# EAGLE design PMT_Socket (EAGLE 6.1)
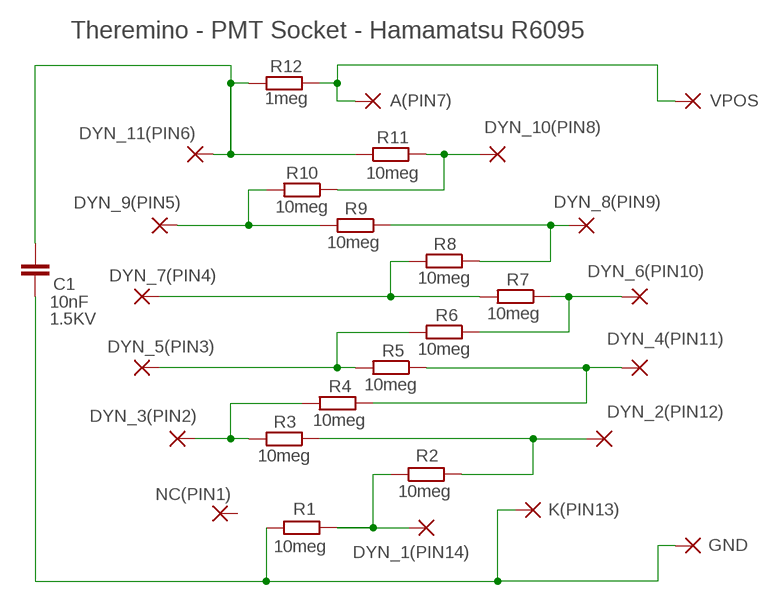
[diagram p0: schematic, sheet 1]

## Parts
A(PIN7)  WIREPAD2,54/1,0  [2,54/1,0]
C1  10nF  C10/4  [C10B4]
DYN_1(PIN14)  WIREPAD2,54/1,0  [2,54/1,0]
DYN_2(PIN12)  WIREPAD2,54/1,0  [2,54/1,0]
DYN_3(PIN2)  WIREPAD2,54/1,0  [2,54/1,0]
DYN_4(PIN11)  WIREPAD2,54/1,0  [2,54/1,0]
DYN_5(PIN3)  WIREPAD2,54/1,0  [2,54/1,0]
DYN_6(PIN10)  WIREPAD2,54/1,0  [2,54/1,0]
DYN_7(PIN4)  WIREPAD2,54/1,0  [2,54/1,0]
DYN_8(PIN9)  WIREPAD2,54/1,0  [2,54/1,0]
DYN_9(PIN5)  WIREPAD2,54/1,0  [2,54/1,0]
DYN_10(PIN8)  WIREPAD2,54/1,0  [2,54/1,0]
DYN_11(PIN6)  WIREPAD2,54/1,0  [2,54/1,0]
GND  WIREPAD2,54/1,0  [2,54/1,0]
K(PIN13)  WIREPAD2,54/1,0  [2,54/1,0]
NC(PIN1)  WIREPAD2,54/1,0  [2,54/1,0]
R1  10meg  R-EU_R1206  [R1206]
R2  10meg  R-EU_R1206  [R1206]
R3  10meg  R-EU_R1206  [R1206]
R4  10meg  R-EU_R1206  [R1206]
R5  10meg  R-EU_R1206  [R1206]
R6  10meg  R-EU_R1206  [R1206]
R7  10meg  R-EU_R1206  [R1206]
R8  10meg  R-EU_R1206  [R1206]
R9  10meg  R-EU_R1206  [R1206]
R10  10meg  R-EU_R1206  [R1206]
R11  10meg  R-EU_R1206  [R1206]
R12  1meg  R-EU_R1206  [R1206]
VPOS  WIREPAD2,54/1,0  [2,54/1,0]

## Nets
N$1: DYN_1(PIN14).1(P) R1.2 R2.1
N$2: C1.1 GND.1(P) K(PIN13).1(P) R1.1
N$3: DYN_2(PIN12).1(P) R2.2 R3.1
N$5: DYN_6(PIN10).1(P) R6.1 R7.1
N$6: DYN_5(PIN3).1(P) R5.2 R6.2
N$7: DYN_4(PIN11).1(P) R4.1 R5.1
N$8: DYN_7(PIN4).1(P) R7.2 R8.2
N$9: DYN_8(PIN9).1(P) R8.1 R9.1
N$10: DYN_10(PIN8).1(P) R10.1 R11.2
N$11: DYN_9(PIN5).1(P) R9.2 R10.2
N$12: C1.2 DYN_11(PIN6).1(P) R11.1 R12.2
N$13: DYN_3(PIN2).1(P) R3.2 R4.2
N$14: A(PIN7).1(P) R12.1 VPOS.1(P)
Unconnected: NC(PIN1).1(P)

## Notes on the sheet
- Theremino - PMT Socket - Hamamatsu R6095

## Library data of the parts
A(PIN7) DYN_1(PIN14) DYN_2(PIN12) DYN_3(PIN2) DYN_4(PIN11) DYN_5(PIN3) DYN_6(PIN10) DYN_7(PIN4) DYN_8(PIN9) DYN_9(PIN5) DYN_10(PIN8) DYN_11(PIN6) GND K(PIN13) NC(PIN1) VPOS = 00-LIVIO:WIREPAD: Wire PAD connect wire on PCB
C1 = 00-LIVIO:C: CAPACITOR; VOLTAGE: 1.5KV
R1-R12 = 00-LIVIO:R-EU_: RESISTOR, European symbol

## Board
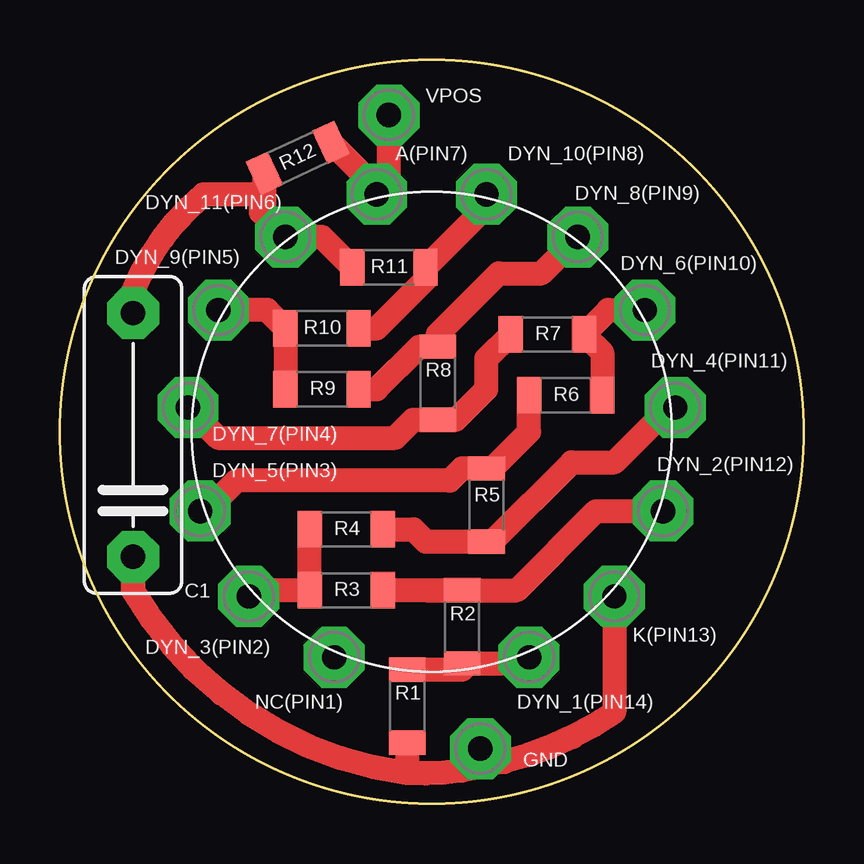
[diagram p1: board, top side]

Size 31 x 31 mm. Coordinates in mm from the lower left corner, seen from the top.
Outline: circle at 15.5,15.5 radius 15.5
Copper layers (1*16): Top 0.035mm / dielectric 1.5mm / Bottom 0.035mm
Design rules: minimum track width 10mil, minimum drill 25mil, track to track 25mil, track to pad 25mil, pad to pad 25mil, via to via 25mil, smd to smd 25mil, copper to edge 25mil, drill to drill 8mil, minimum pad ring 5mil, minimum via ring 8mil, stop-mask expansion 4mil, vias tented up to drill 0mil, thermal gap 38mil

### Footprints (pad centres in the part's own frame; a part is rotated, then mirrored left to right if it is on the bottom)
2,54/1,0 = drill 1.016 pad 2.54 octagon: 1 0,0
C10B4 = drill 1.016 pad 2.159 octagon: 1 -5.08,0; 2 5.08,0
R1206 = smd 1.016 x 1.524: 1 -1.524,0; 2 1.524,0

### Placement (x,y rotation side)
A(PIN7)  13.21,25.4 0 top
C1  3.05,15.37 90 top
DYN_1(PIN14)  19.56,6.1 0 top
DYN_2(PIN12)  25.15,12.19 0 top
DYN_3(PIN2)  7.87,8.64 0 top
DYN_4(PIN11)  25.65,16.51 0 top
DYN_5(PIN3)  5.84,12.19 0 top
DYN_6(PIN10)  24.38,20.57 0 top
DYN_7(PIN4)  5.33,16.51 0 top
DYN_8(PIN9)  21.59,23.62 0 top
DYN_9(PIN5)  6.6,20.57 0 top
DYN_10(PIN8)  17.78,25.4 0 top
DYN_11(PIN6)  9.4,23.62 0 top
GND  17.53,2.29 0 top
K(PIN13)  23.11,8.64 0 top
NC(PIN1)  11.43,6.1 0 top
R1  14.48,4.06 90 top
R2  16.76,7.37 90 top
R3  11.94,8.89 180 top
R4  11.94,11.43 180 top
R5  17.78,12.45 90 top
R6  21.08,17.02 180 top
R7  20.32,19.56 180 top
R8  15.75,17.53 270 top
R9  10.92,17.27 180 top
R10  10.92,19.81 180 top
R11  13.72,22.35 0 top
R12  9.91,26.92 205 top
VPOS  13.72,28.7 0 top

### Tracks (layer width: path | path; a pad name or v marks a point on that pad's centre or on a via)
N$1
  Top 1: 19.56,5.84 R2.1 16.9,5.84 16.9,5.72 16.76,5.59 R1.2 | 19.56,5.84 DYN_1(PIN14).1 19.56,5.84 | 19.56,5.59 19.56,5.84
N$2
  Top 1: K(PIN13).1 23.11,3.81 arc-25 17.53,1.52 | 17.53,1.52 arc-16 14.48,1.27 | 14.48,1.27 arc-52 3.05,8.89 | C1.1 3.05,9.18 | 3.05,9.18 3.05,8.89 | 3.05,8.89 3.05,9.18 | 3.05,9.18 3.05,8.89 | 3.05,8.89 3.05,9.18 | 3.05,9.18 3.05,8.89 | R1.1 14.48,1.27 | GND.1 17.53,1.52
N$3
  Top 1: R2.2 15.24,8.89 | 15.24,8.89 R3.1 | 15.24,8.89 19.05,8.89 22.35,12.19 DYN_2(PIN12).1
N$5
  Top 1: DYN_6(PIN10).1 22.86,20.57 R7.1 22.61,18.8 R6.1
N$6
  Top 1: DYN_5(PIN3).1 6.1,12.19 7.37,13.46 16.26,13.46 16.76,13.97 R5.2 18.03,13.97 19.56,15.49 R6.2
N$7
  Top 1: R4.1 14.73,11.43 15.24,10.92 R5.1 18.03,10.92 21.34,14.22 23.11,14.22 25.4,16.51 DYN_4(PIN11).1
N$8
  Top 1: DYN_7(PIN4).1 6.6,15.24 13.97,15.24 14.73,16 R8.2 16.51,16 17.78,17.27 17.78,18.54 R7.2
N$9
  Top 1: DYN_8(PIN9).1 20.07,22.1 18.29,22.1 18.03,21.84 15.75,19.56 R8.1 15.49,19.05 14.99,19.05 13.21,17.27 R9.1
N$10
  Top 1: DYN_10(PIN8).1 17.78,24.89 R11.2 15.24,21.84 13.21,19.81 R10.1
N$11
  Top 1: DYN_9(PIN5).1 8.64,20.57 R10.2 R9.2
N$12
  Top 1: DYN_11(PIN6).1 8.53,24.5 | 8.53,24.5 R12.2 | C1.2 3.05,21.34 arc-28 5.98,25.4 8.38,25.4 8.38,24.64 DYN_11(PIN6).1 | R11.1 10.92,23.62 DYN_11(PIN6).1 | 8.53,24.5 DYN_11(PIN6).1
N$13
  Top 1: DYN_3(PIN2).1 7.87,8.89 R3.2 R4.2
N$14
  Top 1: R12.1 13.21,25.65 A(PIN7).1 13.72,25.91 VPOS.1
